(* Logix 5000 AddOnInstructionDefinition export SIKO_AP10T; software revision 19.01 *)

ADD_ON_INSTRUCTION SIKO_AP10T   (* revision 5.0 1, vendor SIKO GmbH *)
// SIKO PositionLine AP10T AOI
// Revision note:
// Usable with AP10T Firmware Vers. >= 1.06
VAR_IN_OUT
   DC_OutputBuffer : SINT[10]; {required}
   DC_AbcOutputRegister : AB:ETHERNET_MODULE_SINT_314Bytes:O:0; {required}
END_VAR
VAR_INPUT
   DC_AbcStartByteOut : INT; {required}
END_VAR
VAR_IN_OUT
   DC_InputBuffer : SINT[10]; {required}
   DC_AbcInputRegister : AB:ETHERNET_MODULE_SINT_314Bytes:I:0; {required}
END_VAR
VAR_INPUT
   DC_AbcStartByteIn : INT; {required}
   nNodeId : SINT; {visible}   // Temporaray Node_address
   nSetValue1 : DINT; {visible}
   nSetValue2 : DINT; {visible}
   nParameterAdrRead1 : SINT; {visible}
   nParameterAdrRead2 : SINT; {visible}
   nParameterAdrRead3 : SINT; {visible}
   bcStartRead : BOOL; {visible}
   bcStartWrite : BOOL; {visible}
   bcStartCopy : BOOL; {visible}
   bcResetCounterActivity : BOOL; {visible}
END_VAR
VAR_OUTPUT
   nCounterRead : INT; {access Read Only, visible}
   nCounterWrite : INT; {access Read Only, visible}
   nCounterCopy : INT; {access Read Only, visible}
   nErrorCode1 : SINT; {access Read Only, visible}
   nErrorCode2 : SINT; {access Read Only, visible}
   p00_NodeAddress_r : SINT; {access Read Only, visible}   // Parmeter: 0x00
END_VAR
VAR_INPUT
   p00_NodeAddress_w : SINT; {visible}   // Parmeter: 0x00
END_VAR
VAR_OUTPUT
   p01_Baudrate_r : SINT; {access Read Only}   // Parmeter: 0x01
END_VAR
VAR_INPUT
   p01_Baudrate_w : SINT;   // Parmeter: 0x01
END_VAR
VAR_OUTPUT
   p02_BusTimeout_r : SINT; {access Read Only}   // Parmeter: 0x02
END_VAR
VAR_INPUT
   p02_BusTimeout_w : SINT;   // Parmeter: 0x02
END_VAR
VAR_OUTPUT
   p03_ReplyWriteSetPoint_r : SINT;   // Parmeter: 0x03
END_VAR
VAR_INPUT
   p03_ReplyWriteSetPoint_w : SINT; {access Read Only}   // Parmeter: 0x03
END_VAR
VAR_OUTPUT
   p04_EnableKeysTime_r : SINT; {access Read Only}   // Parmeter: 0x04
END_VAR
VAR_INPUT
   p04_EnableKeysTime_w : SINT;   // Parmeter: 0x04
END_VAR
VAR_OUTPUT
   p05_KeyFunctionEnable1Calibrate_r : SINT; {access Read Only}   // Parmeter: 0x05
END_VAR
VAR_INPUT
   p05_KeyFunctionEnable1Calibrate_w : SINT;   // Parmeter: 0x05
   p06_LedFlashing_w : SINT;   // Parmeter: 0x06
END_VAR
VAR_OUTPUT
   p06_LedFlashing_r : SINT; {access Read Only}   // Parmeter: 0x06
   p08_Led2Red_r : SINT; {access Read Only}   // Parmeter: 0x08
END_VAR
VAR_INPUT
   p08_Led2Red_w : SINT;   // Parmeter: 0x08
END_VAR
VAR_OUTPUT
   p07_Led3Green_r : SINT; {access Read Only}   // Parmeter: 0x07
END_VAR
VAR_INPUT
   p07_Led3Green_w : SINT;   // Parmeter: 0x07
END_VAR
VAR_OUTPUT
   p09_Led1Green_r : SINT; {access Read Only}   // Parmeter: 0x09
END_VAR
VAR_INPUT
   p09_Led1Green_w : SINT;   // Parmeter: 0x09
END_VAR
VAR_OUTPUT
   p0A_DecimalPlaces_r : SINT; {access Read Only}   // Parmeter: 0x0A
END_VAR
VAR_INPUT
   p0A_DecimalPlaces_w : SINT;   // Parmeter: 0x0A
END_VAR
VAR_OUTPUT
   p0D_DisplayOrientation_r : SINT; {access Read Only}   // Parmeter: 0x0D
END_VAR
VAR_INPUT
   p0D_DisplayOrientation_w : SINT;   // Parmeter: 0x0D
END_VAR
VAR_OUTPUT
   p0E_ProgrammingMode_r : SINT; {access Read Only}   // Parmeter: 0x0E
END_VAR
VAR_INPUT
   p0E_ProgrammingMode_w : SINT; {access Read Only}   // Parmeter: 0x0E
END_VAR
VAR_OUTPUT
   p39_Led4Red_r : SINT; {access Read Only}   // Parmeter: 0x39
END_VAR
VAR_INPUT
   p39_Led4Red_w : SINT;   // Parmeter: 0x39
END_VAR
VAR_OUTPUT
   p3A_LcdBacklightFlashing_r : SINT; {access Read Only}   // Parmeter: 0x3A
END_VAR
VAR_INPUT
   p3A_LcdBacklightFlashing_w : SINT;   // Parmeter: 0x3A
END_VAR
VAR_OUTPUT
   p3B_LcdBacklightWhite_r : SINT; {access Read Only}   // Parmeter: 0x3B
END_VAR
VAR_INPUT
   p3B_LcdBacklightWhite_w : SINT;   // Parmeter: 0x3B
END_VAR
VAR_OUTPUT
   p3C_LcdBacklightRed_r : SINT; {access Read Only}   // Parmeter: 0x3C
END_VAR
VAR_INPUT
   p3C_LcdBacklightRed_w : SINT;   // Parmeter: 0x3C
END_VAR
VAR_OUTPUT
   p3D_KeyFunctionEnable3Config_r : SINT; {access Read Only}   // Parmeter: 0x3D
END_VAR
VAR_INPUT
   p3D_KeyFunctionEnable3Config_w : SINT;   // Parmeter: 0x3D
END_VAR
VAR_OUTPUT
   p3E_AcknowledgementSettings_r : SINT; {access Read Only}   // Parmeter: 0x3E
END_VAR
VAR_INPUT
   p3E_AcknowledgementSettings_w : SINT;   // Parmeter: 0x3E
END_VAR
VAR_OUTPUT
   p65_DeviceCode_r : INT; {access Read Only}   // Parmeter: 0x65
   p67_SoftwareVersion_r : INT; {access Read Only}   // Parmeter: 0x67
   p80_NumberOfErrorsRecorded_r : SINT; {access Read Only}   // Parmeter: 0x80
   p81_Error01_r : SINT; {access Read Only}   // Parmeter: 0x81
   p82_Error02_r : SINT; {access Read Only}   // Parmeter: 0x82
   p83_Error03_r : SINT; {access Read Only}   // Parmeter: 0x83
   p84_Error04_r : SINT; {access Read Only}   // Parmeter: 0x84
   p85_Error05_r : SINT; {access Read Only}   // Parmeter: 0x85
   p86_Error06_r : SINT; {access Read Only}   // Parmeter: 0x86
   p87_Error07_r : SINT; {access Read Only}   // Parmeter: 0x87
   p88_Error08_r : SINT; {access Read Only}   // Parmeter: 0x88
   p89_Error09_r : SINT; {access Read Only}   // Parmeter: 0x89
   p8A_Error10_r : SINT; {access Read Only}   // Parmeter: 0x8A
   p96_InputErrors_00_r : INT; {access Read Only}   // Parmeter: 0x96
   p96_InputErrors_01_r : INT; {access Read Only}   // Parmeter: 0x96_Sub1
   p96_InputErrors_02_r : INT; {access Read Only}   // Parmeter: 0x96_Sub2
   p96_InputErrors_03_r : INT; {access Read Only}   // Parmeter: 0x96_Sub3
   p96_InputErrors_04_r : INT; {access Read Only}   // Parmeter: 0x96_Sub4
   p96_InputErrors_05_r : INT; {access Read Only}   // Parmeter: 0x96_Sub5
   p96_InputErrors_06_r : INT; {access Read Only}   // Parmeter: 0x96_Sub6
   p96_InputErrors_07_r : INT; {access Read Only}   // Parmeter: 0x96_Sub7
   p96_InputErrors_08_r : INT; {access Read Only}   // Parmeter: 0x96_Sub8
   p96_InputErrors_09_r : INT; {access Read Only}   // Parmeter: 0x96_Sub9
   p96_InputErrors_10_r : INT; {access Read Only}   // Parmeter: 0x96_Sub10
END_VAR
VAR_INPUT
   pA0_SystemCommand_w : SINT;   // Parmeter: 0xA0
   pA8_ProgrammingModeOnOff_w : SINT;   // Parmeter: 0xA8
END_VAR
VAR_OUTPUT
   pD0_ResponseDelay_r : SINT; {access Read Only}   // Parmeter: 0xD0
END_VAR
VAR_INPUT
   pD0_ResponseDelay_w : SINT;   // Parmeter: 0xD0
   pD2_AutoIdAssignment_w : SINT;   // Parmeter: 0xD2
END_VAR
VAR_OUTPUT
   pFA_SystemStatusword_r : INT; {access Read Only}   // Parmeter: 0xFA
   pFB_SetPoint1_r : DINT; {access Read Only}   // Parmeter: 0xFB
   pFF_SetPoint2_r : DINT; {access Read Only}   // Parmeter: 0xFF
END_VAR
VAR_INPUT
   bc02_ValidityOfSetpoint1 : BOOL;
   bc03_DisplayRange : BOOL;
   bc05_ErrorAcknowledgment : BOOL;
   bc06_AcknowledgementOfSetpoint2 : BOOL;
   bc07_DataIdentifier : BOOL;
   bc09_ValidityOfSetpoint2 : BOOL;
   bc10_AcknowledgementOfSetpoint1 : BOOL;
   bc11_Led1GreenLeft : BOOL;
   bc12_Led3GreenRight : BOOL;
   bc13_Led4RedRight : BOOL;
   bc14_Led2RedLeft : BOOL;
   bc15_LedBlinking : BOOL;
END_VAR
VAR_OUTPUT
   bs02_ValiditySetpoint1 : BOOL; {access Read Only}
   bs03_AcknowledgementOfSetpoint2 : BOOL; {access Read Only}
   bs05_AcknowledgementOfSetpoint1 : BOOL; {access Read Only}
   bs06_Deviation : BOOL; {access Read Only}
   bs07_DeviceError : BOOL; {access Read Only}
   bs08_ButtonFront : BOOL; {access Read Only}
   bs09_DataIdentifier : BOOL; {access Read Only}
   bs10_ValiditySetpoint2 : BOOL;
   bs13_ButtonLeft : BOOL; {access Read Only}
   bs14_ButtonStar : BOOL; {access Read Only}
   bs15_ButtonUp : BOOL; {access Read Only}
   bsDone : BOOL; {access Read Only, visible}
   bsBusy : BOOL; {access Read Only, visible}
   bsFaultDataReceive : BOOL; {access Read Only, visible}
   bsComTimeout : BOOL; {access Read Only, visible}
   bsGeneralError : BOOL; {access Read Only, visible}
END_VAR
VAR
   vnTriggerTx : SINT; {access None}
   vnCounterToggle : SINT; {access None}
   vnTriggerRx : SINT; {access None}
   vnParameterAdrReceive : INT; {access None}
   vnParameterAdrSend : INT; {access None}
   vnParameterDataReceive : DINT; {access None}
   vnParameterDataSend : DINT; {access None}
   vbRefresh : BOOL; {access None}
   vbOsrWrite : BOOL; {access None}
   vbOsrRead : BOOL; {access None}
   vnOutputDataOffset : DINT; {access None}
   vnDcOutputBufferTemp : DINT; {access None}
   vnDcInputBufferTemp : DINT; {access None}
   vbOsrCopy : BOOL; {access None}
   SN5_ABC : FBD_TIMER; {access None}
END_VAR

ROUTINE Logic   (* structured text *)
   ///////////////////////////////////////////////////////////////////////////////////////////////
   // Name:	SIKO_AP10T
   ///////////////////////////////////////////////////////////////////////////////////////////////
   // Version history
   ///////////////////////////////////////////////////////////////////////////////////////////////
   // Date        | Version  | created under          	| Author    		| Remark
   // dd.mm.yyyy  | 		  |							|					|
   // -----------------------------------------------------------------------------------
   // 07.09.2015  | 5.0.1    | V19.01.00 (CPR 9 SR 3)  | SIKO GmbH / SC 	| basic version
   ///////////////////////////////////////////////////////////////////////////////////////////////
   
   ///////////////////////////////////////////////////////////////////////////////////////////////
   // Init at first scan
   //
   IF s:fs THEN
   	bcStartRead :=0;
   	bcStartWrite :=0;
   	bcStartCopy :=0;
   	nCounterCopy := 0;
   	nCounterWrite := 0;
   	nCounterRead := 0;
   	vnCounterToggle := 0;
   	bcResetCounterActivity := 0;
   END_IF;
   
   ///////////////////////////////////////////////////////////////////////////////////////////////
   // read inputs synchonous
   //
   CPS(DC_AbcInputRegister.data[DC_AbcStartByteIn] , DC_InputBuffer[0],10); // read from ABC
   
   ///////////////////////////////////////////////////////////////////////////////////////////////
   // input byte swop to parameter data and format transfer vnParameterAdrReceive
   //
   cop (DC_InputBuffer[5], vnDcInputBufferTemp, 1);					//Data Type Conversion
   swpb (vnDcInputBufferTemp, Reverse, vnParameterDataReceive);
   
   vnParameterAdrReceive := 16#00ff and DC_InputBuffer[2];
   
   ///////////////////////////////////////////////////////////////////////////////////////////////
   // New telegram arrived in time
   //
   SN5_ABC.Pre := (p02_BusTimeout_r * 100) + 500;							// 2000 milliseconds
   SN5_ABC.Reset := vnTriggerRx <> DC_InputBuffer[9];
   SN5_ABC.TimerEnable := vnTriggerRx = DC_InputBuffer[9];
   RTOR(SN5_ABC);
   bsComTimeout := SN5_ABC.DN;
   
   vnTriggerRx:= DC_InputBuffer[9]; // Trigger received
   
   ///////////////////////////////////////////////////////////////////////////////////////////////
   // Telegram acknowledge checked for bad reply
   //
   if vnParameterAdrReceive = 253
   then
   	bsFaultDataReceive := 1;
   	nErrorCode1 := DC_InputBuffer[8];
   	nErrorCode2 := DC_InputBuffer[7];
   
   else
   	bsFaultDataReceive := 0;
   	nErrorCode1 := 0;
   	nErrorCode2 := 0;
   end_if;
   
   
   ///////////////////////////////////////////////////////////////////////////////////////////////
   // Request (Read/Write) successful
   //
   if DC_OutputBuffer[2] = DC_InputBuffer[2] and not bsFaultDataReceive
   then
   	if nCounterRead <> 0
   	then
   		if vnParameterAdrReceive = 150							// check for parameter 0x96 Input Errors and Indexrutine
   		then
   			if DC_OutputBuffer[5] = DC_InputBuffer[5]			// check for Index: DataSend = DataReceive
   			then
   				nCounterRead := nCounterRead + 1;
   			end_if;
   		else
   			nCounterRead := nCounterRead + 1;
   		end_if;
   	end_if;
   	if nCounterWrite <> 0
   	then
   		nCounterWrite := nCounterWrite + 1;
   	end_if;
   end_if;
   
   ///////////////////////////////////////////////////////////////////////////////////////////////
   // Control word
   //
   DC_OutputBuffer[4].0 := 0;
   DC_OutputBuffer[4].1 := 0;
   DC_OutputBuffer[4].2 := bc02_ValidityOfSetpoint1;                // Validity of setpoint1; 0=invalid; 1=valid
   DC_OutputBuffer[4].3 := bc03_DisplayRange;                       // Display range full
   DC_OutputBuffer[4].4 := 0;
   DC_OutputBuffer[4].5 := bc05_ErrorAcknowledgment;                // Acknowledged
   DC_OutputBuffer[4].6 := bc06_AcknowledgementOfSetpoint2;         // Acknowledgment Set Value2
   DC_OutputBuffer[4].7 := bc07_DataIdentifier;                     // Data format, Number / ASCII-String
   DC_OutputBuffer[3].0 := 0;
   DC_OutputBuffer[3].1 := bc09_ValidityOfSetpoint2;                // Validity of setpoint2
   DC_OutputBuffer[3].2 := bc10_AcknowledgementOfSetpoint1;         // Acknowledgment Set Value2
   DC_OutputBuffer[3].3 := bc11_Led1GreenLeft;                      // LED1 green left
   DC_OutputBuffer[3].4 := bc12_Led3GreenRight;                     // LED3 green right
   DC_OutputBuffer[3].5 := bc13_Led4RedRight;                       // LED4 red right
   DC_OutputBuffer[3].6 := bc14_Led2RedLeft;                        // LED2 red left
   DC_OutputBuffer[3].7 := bc15_LedBlinking;                        // LED blinking
   
   ///////////////////////////////////////////////////////////////////////////////////////////////
   // Start Read
   //
   IF (bcStartRead or vbRefresh) AND (nCounterRead = 0) AND (nCounterWrite = 0) AND (nCounterCopy = 0)  AND NOT vbOsrRead
   THEN
   	nCounterRead := 1;
   	nCounterWrite := 0;
   	nCounterCopy := 0;
   	vbRefresh := 0;
   	vbOsrRead := 1;
   END_IF;
   IF NOT bcStartRead and vbOsrRead
   THEN
   	vbOsrRead := 0;
   END_IF;
   
   ///////////////////////////////////////////////////////////////////////////////////////////////
   // Start Write
   //
   IF bcStartWrite AND (nCounterRead = 0) AND (nCounterWrite = 0) AND (nCounterCopy = 0) AND NOT vbOsrWrite
   THEN
   	nCounterWrite := 1;
   	nCounterRead := 0;
   	nCounterCopy := 0;
   	vbOsrWrite := 1;
   END_IF;
   IF NOT bcStartWrite and vbOsrWrite
   THEN
   	vbOsrWrite := 0;
   END_IF;
   
   ///////////////////////////////////////////////////////////////////////////////////////////////
   // copy read to write parameters
   //
   IF bcStartCopy AND (nCounterRead = 0) AND (nCounterWrite = 0) AND (nCounterCopy = 0) AND NOT vbOsrCopy
   THEN
   	nCounterCopy := 1;
   	nCounterWrite := 0;
   	nCounterRead := 0;
   	vbOsrCopy := 1;
   END_IF;
   IF NOT bcStartCopy and vbOsrCopy
   THEN
   	vbOsrCopy := 0;
   END_IF;
   
   ///////////////////////////////////////////////////////////////////////////////////////////////
   // reset counter (nCounter...) and activity (bcStart...)
   //
   IF bcResetCounterActivity
   THEN
   	bcStartRead :=0;
   	bcStartWrite :=0;
   	bcStartCopy :=0;
   	nCounterCopy := 0;
   	nCounterWrite := 0;
   	nCounterRead := 0;
   	vnCounterToggle := 0;
   	bcResetCounterActivity := 0;
   END_IF;
   
   ///////////////////////////////////////////////////////////////////////////////////////////////
   // Parameter request
   //
   if nCounterRead > 0
   	then
   	DC_OutputBuffer[0] := 0;
   	vnParameterDataSend := 0;
   	CASE nCounterRead OF
   	1: //0x00 Note address
   	    vnParameterAdrSend := 0;
   	2: //0x01 Baud rate
   		vnParameterAdrSend := 1;
   	3: //0x02 Bus Timeout
         	vnParameterAdrSend := 2;
   	4: //0x03 Response parameter to a setpoint write access
         	vnParameterAdrSend := 3;
   	5: //0x04 Keys enable time: Configuration start delay
         	vnParameterAdrSend := 4;
   	6: //0x05 Key function enable1: Calibration enable
         	vnParameterAdrSend := 5;
   	7: //0x06 LED flashing
         	vnParameterAdrSend := 6;
   	8: //0x07 LED3 (green right)
         	vnParameterAdrSend := 7;
   	9: //0x08 LED2 (red left)
         	vnParameterAdrSend := 8;
   	10: //0x09 LED1 (green left)
         	vnParameterAdrSend := 9;
   	11: //0x0A Decimal places
         	vnParameterAdrSend := 10;
   	12: //0x0D Display orientation
         	vnParameterAdrSend := 13;
   	13: //0x0E Configuration programming mode
         	vnParameterAdrSend := 14;
   	14: //0x39 LED4 (red right)
         	vnParameterAdrSend := 57;
   	15: //0x3A LCD backlight flashing
         	vnParameterAdrSend := 58;
   	16: //0x3B LCD backlight white
         	vnParameterAdrSend := 59;
   	17: //0x3C LCD backlight red
         	vnParameterAdrSend := 60;
   	18: //0x3D Key function enable3: Configuration enable via keyboard
         	vnParameterAdrSend := 61;
   	19: //0x3E Acknowledgement settings
         	vnParameterAdrSend := 62;
   	20: //0x65 Device identification
         	vnParameterAdrSend := 101;
   	21: //0x67 Software version
         	vnParameterAdrSend := 103;
   	22: //0x80 Number of errors
         	vnParameterAdrSend := 128;
   	23: //0x81 Error 01
         	vnParameterAdrSend := 129;
   	24: //0x82 Error 02
         	vnParameterAdrSend := 130;
   	25: //0x83 Error 03
         	vnParameterAdrSend := 131;
   	26: //0x84 Error 04
         	vnParameterAdrSend := 132;
   	27: //0x85 Error 05
         	vnParameterAdrSend := 133;
   	28: //0x86 Error 06
         	vnParameterAdrSend := 134;
   	29: //0x87 Error 07
         	vnParameterAdrSend := 135;
   	30: //0x88 Error 08
         	vnParameterAdrSend := 136;
   	31: //0x89 Error 09
         	vnParameterAdrSend := 137;
   	32: //0x8A Error 10
         	vnParameterAdrSend := 138;
   	33: //0x96 Input Errors
   		vnParameterAdrSend := 150;
   	34: //0x96_1 Input Errors Index 1
   		vnParameterAdrSend := 150;
   		vnParameterDataSend := 16#01000000;
   	35: //0x96_2 Input Errors Index 2
   		vnParameterAdrSend := 150;
   		vnParameterDataSend := 16#02000000;
   	36: //0x96_3 Input Errors Index 3
   		vnParameterAdrSend := 150;
   		vnParameterDataSend := 16#03000000;
   	37: //0x96_4 Input Errors Index 4
   		vnParameterAdrSend := 150;
   		vnParameterDataSend := 16#04000000;
   	38: //0x96_5 Input Errors Index 5
   		vnParameterAdrSend := 150;
   		vnParameterDataSend := 16#05000000;
   	39: //0x96_6 Input Errors Index 6
   		vnParameterAdrSend := 150;
   		vnParameterDataSend := 16#06000000;
   	40: //0x96_7 Input Errors Index 7
   		vnParameterAdrSend := 150;
   		vnParameterDataSend := 16#07000000;
   	41: //0x96_8 Input Errors Index 8
   		vnParameterAdrSend := 150;
   		vnParameterDataSend := 16#08000000;
   	42: //0x96_9 Input Errors Index 9
   		vnParameterAdrSend := 150;
   		vnParameterDataSend := 16#09000000;
   	43: //0x96_10 Input Errors Index 10
   		vnParameterAdrSend := 150;
   		vnParameterDataSend := 16#0A000000;
   	44: //0xD0 Response delay
         	vnParameterAdrSend := 208;
   	45: //0xFA System Status word
         	vnParameterAdrSend := 250;
   	46: //0xFB Setpoint1
         	vnParameterAdrSend := 251;
   	47: //0xFF Setpoint2
         	vnParameterAdrSend := 255;
   	48: // Parameter read completed
   		nCounterRead := 0;
     	END_CASE;
   end_if;
   
   ///////////////////////////////////////////////////////////////////////////////////////////////
   // Parameter Settings
   //
   if nCounterWrite > 0
   	then
   	DC_OutputBuffer[0] := 1;
   	CASE nCounterWrite OF
   	1: //Programming mode
   		IF pA8_ProgrammingModeOnOff_w >= 0 and pA8_ProgrammingModeOnOff_w <= 1
   		THEN
   	      	vnParameterAdrSend := 168;
   			vnParameterDataSend:= pA8_ProgrammingModeOnOff_w;
   		END_IF;
   	2: //Note address
   		IF p00_NodeAddress_w <> p00_NodeAddress_r or bsFaultDataReceive
   		THEN
   	      	vnParameterAdrSend := 0;
   			vnParameterDataSend:= p00_NodeAddress_w;
   		END_IF;
   	3: //Baudrate
   		IF p01_Baudrate_w <> p01_Baudrate_r or bsFaultDataReceive
   		THEN
   	      	vnParameterAdrSend := 1;
   			vnParameterDataSend:= p01_Baudrate_w;
   		END_IF;
   	4: //Bus Timeout
   		IF p02_BusTimeout_w <> p02_BusTimeout_r or bsFaultDataReceive
   		THEN
   	      	vnParameterAdrSend := 2;
   			vnParameterDataSend:= p02_BusTimeout_w;
   		END_IF;
   	5: //Response parameter to a setpoint write access
   		IF p03_ReplyWriteSetPoint_w <> p03_ReplyWriteSetPoint_r or bsFaultDataReceive
   		THEN
   	      	vnParameterAdrSend := 3;
   			vnParameterDataSend:= p03_ReplyWriteSetPoint_w;
   		END_IF;
   	6: ///Keys enable time: Configuration start delay
   		IF p04_EnableKeysTime_w <> p04_EnableKeysTime_r or bsFaultDataReceive
   		THEN
   	      	vnParameterAdrSend := 4;
   			vnParameterDataSend:= p04_EnableKeysTime_w;
   		END_IF;
   	7: //Key function enable1: Calibration enable
   		IF p05_KeyFunctionEnable1Calibrate_w <> p05_KeyFunctionEnable1Calibrate_r or bsFaultDataReceive
   		THEN
   	      	vnParameterAdrSend := 5;
   			vnParameterDataSend:= p05_KeyFunctionEnable1Calibrate_w;
   		END_IF;
   	8: //LED flashing
   		IF p06_LedFlashing_w <> p06_LedFlashing_r or bsFaultDataReceive
   		THEN
   	      	vnParameterAdrSend := 6;
   			vnParameterDataSend:= p06_LedFlashing_w;
   		END_IF;
   	9: //LED3 (green right)
   		IF p07_Led3Green_w <> p07_Led3Green_r or bsFaultDataReceive
   		THEN
   	      	vnParameterAdrSend := 7;
   			vnParameterDataSend:= p07_Led3Green_w;
   		END_IF;
   	10: //LED2 (red left)
   		IF p08_Led2Red_w <> p08_Led2Red_r or bsFaultDataReceive
   		THEN
   	      	vnParameterAdrSend := 8;
   			vnParameterDataSend:= p08_Led2Red_w;
   		END_IF;
   	11: //LED1 (green left)
   		IF p09_Led1Green_w <> p09_Led1Green_r or bsFaultDataReceive
   		THEN
   	      	vnParameterAdrSend := 9;
   			vnParameterDataSend:= p09_Led1Green_w;
   		END_IF;
   	12: //Decimal places
   		IF p0A_DecimalPlaces_w <> p0A_DecimalPlaces_r or bsFaultDataReceive
   		THEN
   	      	vnParameterAdrSend := 10;
   			vnParameterDataSend := p0A_DecimalPlaces_w;
   		END_IF;
   	13: //Display orientation
   		IF p0D_DisplayOrientation_w <> p0D_DisplayOrientation_r or bsFaultDataReceive
   		THEN
   	      	vnParameterAdrSend := 13;
   			vnParameterDataSend:= p0D_DisplayOrientation_w;
   		END_IF;
   	14: //Configuration programming mode
   		IF p0E_ProgrammingMode_w <> p0E_ProgrammingMode_r or bsFaultDataReceive
   		THEN
   	      	vnParameterAdrSend := 14;
   			vnParameterDataSend:= p0E_ProgrammingMode_w;
   		END_IF;
   	15: //LED4 (red right)
   		IF p39_Led4Red_w <> p39_Led4Red_r or bsFaultDataReceive
   		THEN
   	      	vnParameterAdrSend := 57;
   			vnParameterDataSend:= p39_Led4Red_w;
   		END_IF;
   	16: //LCD backlight flashing
   		IF p3A_LcdBacklightFlashing_w <> p3A_LcdBacklightFlashing_r or bsFaultDataReceive
   		THEN
   	      	vnParameterAdrSend := 58;
   			vnParameterDataSend:= p3A_LcdBacklightFlashing_w;
   		END_IF;
   	17: //LCD backlight white
   		IF p3B_LcdBacklightWhite_w <> p3B_LcdBacklightWhite_r or bsFaultDataReceive
   		THEN
   	      	vnParameterAdrSend := 59;
   			vnParameterDataSend:= p3B_LcdBacklightWhite_w;
   		END_IF;
   	18: //LCD backlight red
   		IF p3C_LcdBacklightRed_w <> p3C_LcdBacklightRed_r or bsFaultDataReceive
   		THEN
   	      	vnParameterAdrSend := 60;
   			vnParameterDataSend:= p3C_LcdBacklightRed_w;
   		END_IF;
   	19: //Key function enable3: Configuration enable via keyboard
   		IF p3D_KeyFunctionEnable3Config_w <> p3D_KeyFunctionEnable3Config_r or bsFaultDataReceive
   		THEN
   	      	vnParameterAdrSend := 61;
   			vnParameterDataSend:= p3D_KeyFunctionEnable3Config_w;
   		END_IF;
   	20: //Acknowledgement settings
   		IF p3E_AcknowledgementSettings_w <> p3E_AcknowledgementSettings_r or bsFaultDataReceive
   		THEN
   	      	vnParameterAdrSend := 62;
   			vnParameterDataSend:= p3E_AcknowledgementSettings_w;
   		END_IF;
   	21: //Response delay
   		IF pD0_ResponseDelay_w <> pD0_ResponseDelay_r or bsFaultDataReceive
   		THEN
   	      	vnParameterAdrSend := 208;
   			vnParameterDataSend:= pD0_ResponseDelay_w;
   		END_IF;
   	22: //Auto-ID assignment
   		IF pD2_AutoIdAssignment_w >= 1 and pD2_AutoIdAssignment_w <= 31 and nNodeId = 31
   		THEN
   	      	vnParameterAdrSend := 210;
   			vnParameterDataSend:= pD2_AutoIdAssignment_w;
   		END_IF;
   	23: //S-Befehl
   		IF pA0_SystemCommand_w >= 1 and pA0_SystemCommand_w <= 9 // check, if value is between 1 and 9
   		THEN
   	      	vnParameterAdrSend := 160;
   			vnParameterDataSend:= pA0_SystemCommand_w;
   			vbRefresh := 1;
   		END_IF;
   	24:	//Write complete start refresh if S-Command
   		nCounterWrite := 0;
   
   	END_CASE;
   end_if;
   ///////////////////////////////////////////////////////////////////////////////////////////////
   // Read/Write standard values and three free parameters if parameter read/write inactive
   //
   if (nCounterRead = 0) and (nCounterWrite = 0)
   then
   	if (vnCounterToggle < 1) or (vnCounterToggle > 5)
   	then
   		vnCounterToggle := 1;
   	end_if;
   
   	CASE vnCounterToggle OF
   	1:	//check SetValue and transmit
   		DC_OutputBuffer[0] := 1;
      		vnParameterAdrSend := 251;
   		vnParameterDataSend := nSetValue1;
   
   		if (vnParameterAdrReceive = 251) and DC_InputBuffer[0] = 1
   		then
   			vnCounterToggle := vnCounterToggle + 1;
   		end_if;
   
   	2:	//check SetValue and transmit
   		DC_OutputBuffer[0] := 1;
      		vnParameterAdrSend := 255;
   		vnParameterDataSend := nSetValue2;
   
   		if (vnParameterAdrReceive = 255) and DC_InputBuffer[0] = 1
   		then
   			vnCounterToggle := vnCounterToggle + 1;
   		end_if;
   
   	3:	//vnParameterAdrRead1
   		if ((16#00ff and nParameterAdrRead1) <= 250)
   		then
   			DC_OutputBuffer[0] := 0;
   			vnParameterAdrSend := nParameterAdrRead1;
   			vnParameterDataSend := 0;
   		else
   			vnCounterToggle := vnCounterToggle + 1;
   		end_if;
   
   		if vnParameterAdrReceive = (16#00ff and nParameterAdrRead1) and DC_InputBuffer[0] = 0
   		then
   			vnCounterToggle := vnCounterToggle + 1;
   		end_if;
   
   	4:	//vnParameterAdrRead2
   		if ((16#00ff and nParameterAdrRead2) <= 250)
   		then
   			DC_OutputBuffer[0] := 0;
   			vnParameterAdrSend := nParameterAdrRead2;
   			vnParameterDataSend := 0;
   		else
   			vnCounterToggle := vnCounterToggle + 1;
   		end_if;
   
   		if vnParameterAdrReceive = (16#00ff and nParameterAdrRead2) and DC_InputBuffer[0] = 0
   		then
   			vnCounterToggle := vnCounterToggle + 1;
   		end_if;
   
   	5:	//vnParameterAdrRead3
   		if ((16#00ff and nParameterAdrRead3) <= 250)
   		then
   			DC_OutputBuffer[0] := 0;
   			vnParameterAdrSend := nParameterAdrRead3;
   			vnParameterDataSend := 0;
   		else
   			vnCounterToggle := vnCounterToggle + 1;
   		end_if;
   
   		if vnParameterAdrReceive = (16#00ff and nParameterAdrRead3) and DC_InputBuffer[0] = 0
   		then
   			vnCounterToggle := vnCounterToggle + 1;
   		end_if;
   
   	END_CASE;
   else
   	vnCounterToggle := 0;
   end_if;
   
   ///////////////////////////////////////////////////////////////////////////////////////////////
   // Because of Arthmetic overflow
   //
   if vnTriggerTx >= 127
   then
    vnTriggerTx := -128;
   end_if;
   vnTriggerTx := vnTriggerTx + 1; // ABC Update mode: Change of state on trigger
   
   ///////////////////////////////////////////////////////////////////////////////////////////////
   // Telegram will be completed
   //
   DC_OutputBuffer[1] := nNodeId;
   DC_OutputBuffer[2] := 16#00ff and vnParameterAdrSend;
   DC_OutputBuffer[9] := vnTriggerTx; // Trigger transmit
   
   ///////////////////////////////////////////////////////////////////////////////////////////////
   ///////////////////////////////////////////////////////////////////////////////////////////////
   
   ///////////////////////////////////////////////////////////////////////////////////////////////
   // Confirmation of Parameter request / Parameter Settings
   //
   IF DC_InputBuffer[1] = nNodeId //Check node address
   THEN
   //	vnParameterAdrReceive := 16#00ff and DC_InputBuffer[2]; //Check command acknowledgment
   	CASE vnParameterAdrReceive OF
   		251: //Setpoint1
   			COP (vnParameterDataReceive,pFB_SetPoint1_r,1);
   		255: //Setpoint2
   			COP (vnParameterDataReceive,pFF_SetPoint2_r,1);
   		0: //Note address
   			COP (vnParameterDataReceive,p00_NodeAddress_r,1);
   		1: //Baudrate
   			COP (vnParameterDataReceive,p01_Baudrate_r,1);
   		2: //Bus Timeout
   			COP (vnParameterDataReceive,p02_BusTimeout_r,1);
   		3: //Response parameter to a setpoint write access
   			COP (vnParameterDataReceive,p03_ReplyWriteSetPoint_r,1);
   		4: //Keys enable time: Configuration start delay
   			COP (vnParameterDataReceive,p04_EnableKeysTime_r,1);
   		5: //Key function enable1: Calibration enable
   			COP (vnParameterDataReceive,p05_KeyFunctionEnable1Calibrate_r,1);
   		6: //LED flashing
   			COP (vnParameterDataReceive,p06_LedFlashing_r,1);
   		7: //LED3 (green right)
   			COP (vnParameterDataReceive,p07_Led3Green_r,1);
   		8: //LED2 (red left)
   			COP (vnParameterDataReceive,p08_Led2Red_r,1);
   		9: //LED1 (green left)
   			COP (vnParameterDataReceive,p09_Led1Green_r,1);
   		10: //Decimal places
   			COP (vnParameterDataReceive,p0A_DecimalPlaces_r,1);
   		13: //Display orientation
   			COP (vnParameterDataReceive,p0D_DisplayOrientation_r,1);
   		14: //Configuration programming mode
   			COP (vnParameterDataReceive,p0E_ProgrammingMode_r,1);
   		57:	//LED4 (red right)
   			COP (vnParameterDataReceive,p39_Led4Red_r,1);
   		58:	//LCD backlight flashing
   			COP (vnParameterDataReceive,p3A_LcdBacklightFlashing_r,1);
   		59:	//LCD backlight white
   			COP (vnParameterDataReceive,p3B_LcdBacklightWhite_r,1);
   		60:	//LCD backlight red
   			COP (vnParameterDataReceive,p3C_LcdBacklightRed_r,1);
   		61: //Key function enable3: Configuration enable via keyboard
   			COP (vnParameterDataReceive,p3D_KeyFunctionEnable3Config_r,1);
   		62:	//Acknowledgement settings
   			COP (vnParameterDataReceive,p3E_AcknowledgementSettings_r,1);
   		101: //Device identification
   			COP (vnParameterDataReceive,p65_DeviceCode_r,1);
   		103: //Software version
   			COP (vnParameterDataReceive,p67_SoftwareVersion_r,1);
   		128: //Number of errors
   			COP (vnParameterDataReceive,p80_NumberOfErrorsRecorded_r,1);
   		129: //Error01
   			COP (vnParameterDataReceive,p81_Error01_r,1);
   		130: //Error02
   			COP (vnParameterDataReceive,p82_Error02_r,1);
   		131: //Error03
   			COP (vnParameterDataReceive,p83_Error03_r,1);
   		132: //Error04
   			COP (vnParameterDataReceive,p84_Error04_r,1);
   		133: //Error05
   			COP (vnParameterDataReceive,p85_Error05_r,1);
   		134: //Error06
   			COP (vnParameterDataReceive,p86_Error06_r,1);
   		135: //Error07
   			COP (vnParameterDataReceive,p87_Error07_r,1);
   		136: //Error08
   			COP (vnParameterDataReceive,p88_Error08_r,1);
   		137: //Error09
   			COP (vnParameterDataReceive,p89_Error09_r,1);
   		138: //Error10
   			COP (vnParameterDataReceive,p8A_Error10_r,1);
   		150: //Input errors
   			if vnParameterDataSend = 0
   				then
   					COP (vnParameterDataReceive,p96_InputErrors_00_r,1);
   				end_if;
   			if vnParameterDataSend = 16#01000000
   				then
   					COP (vnParameterDataReceive,p96_InputErrors_01_r,1);
   				end_if;
   			if vnParameterDataSend = 16#02000000
   				then
   					COP (vnParameterDataReceive,p96_InputErrors_02_r,1);
   				end_if;
   			if vnParameterDataSend = 16#03000000
   				then
   					COP (vnParameterDataReceive,p96_InputErrors_03_r,1);
   				end_if;
   			if vnParameterDataSend = 16#04000000
   				then
   					COP (vnParameterDataReceive,p96_InputErrors_04_r,1);
   				end_if;
   			if vnParameterDataSend = 16#05000000
   				then
   					COP (vnParameterDataReceive,p96_InputErrors_05_r,1);
   				end_if;
   			if vnParameterDataSend = 16#06000000
   				then
   					COP (vnParameterDataReceive,p96_InputErrors_06_r,1);
   				end_if;
   			if vnParameterDataSend = 16#07000000
   				then
   					COP (vnParameterDataReceive,p96_InputErrors_07_r,1);
   				end_if;
   			if vnParameterDataSend = 16#08000000
   				then
   					COP (vnParameterDataReceive,p96_InputErrors_08_r,1);
   				end_if;
   			if vnParameterDataSend = 16#09000000
   				then
   					COP (vnParameterDataReceive,p96_InputErrors_09_r,1);
   				end_if;
   			if vnParameterDataSend = 16#0A000000
   				then
   					COP (vnParameterDataReceive,p96_InputErrors_10_r,1);
   				end_if;
   
   		208: //Response delay
   			COP (vnParameterDataReceive,pD0_ResponseDelay_r,1);
   		250: //System Status word
   			COP (vnParameterDataReceive,pFA_SystemStatusword_r,1);
   		END_CASE;
   END_IF;
   
   ///////////////////////////////////////////////////////////////////////////////////////////////
   // handle copy instruction
   //
   
   IF (nCounterCopy > 0)
   THEN
   	p00_NodeAddress_w := p00_NodeAddress_r;
   	p01_Baudrate_w := p01_Baudrate_r;
   	p02_BusTimeout_w := p02_BusTimeout_r;
   	p03_ReplyWriteSetPoint_w := p03_ReplyWriteSetPoint_r;
   	p04_EnableKeysTime_w := p04_EnableKeysTime_r;
   	p05_KeyFunctionEnable1Calibrate_w := p05_KeyFunctionEnable1Calibrate_r;
   	p06_LedFlashing_w := p06_LedFlashing_r;
   	p07_Led3Green_w := p07_Led3Green_r;
   	p08_Led2Red_w := p08_Led2Red_r;
   	p09_Led1Green_w := p09_Led1Green_r;
   	p0A_DecimalPlaces_w := p0A_DecimalPlaces_r;
   	p0D_DisplayOrientation_w := p0D_DisplayOrientation_r;
   	p0E_ProgrammingMode_w := p0E_ProgrammingMode_r;
   	p39_Led4Red_w := p39_Led4Red_r;
   	p3A_LcdBacklightFlashing_w := p3A_LcdBacklightFlashing_r;
   	p3B_LcdBacklightWhite_w := p3B_LcdBacklightWhite_r;
   	p3C_LcdBacklightRed_w := p3C_LcdBacklightRed_r;
   	p3D_KeyFunctionEnable3Config_w := p3D_KeyFunctionEnable3Config_r;
   	p3E_AcknowledgementSettings_w := p3E_AcknowledgementSettings_r;
   	pD0_ResponseDelay_w := pD0_ResponseDelay_r;
   
   	nCounterCopy := 0;
   END_IF;
   
   ///////////////////////////////////////////////////////////////////////////////////////////////
   // Status word
   //
   // bs00_ 				 					:= DC_InputBuffer[4].0;
   // bs01_									:= DC_InputBuffer[4].1;
   bs02_ValiditySetpoint1 						:= DC_InputBuffer[4].2; //set_value1_ack
   bs03_AcknowledgementOfSetpoint2				:= DC_InputBuffer[4].3; //AcknowledgementOfSetpoint2
   // bs04_									:= DC_InputBuffer[4].4;
   bs05_AcknowledgementOfSetpoint1				:= DC_InputBuffer[4].5; //AcknowledgementOfSetpoint1
   bs06_Deviation								:= DC_InputBuffer[4].6; //deviation
   bs07_DeviceError 							:= DC_InputBuffer[4].7; //Error
   bs08_ButtonFront		 					:= DC_InputBuffer[3].0; //AV_position
   bs09_DataIdentifier							:= DC_InputBuffer[3].1; //incremental_measure
   bs10_ValiditySetpoint2          			:= DC_InputBuffer[3].2; //set_value2_ack
   // bs11_			 						:= DC_InputBuffer[3].3;
   // bs12_			           				:= DC_InputBuffer[3].4;
   bs13_ButtonLeft 							:= DC_InputBuffer[3].5; //button_left
   bs14_ButtonStar 							:= DC_InputBuffer[3].6; //button_star
   bs15_ButtonUp 								:= DC_InputBuffer[3].7; //button_up
   
   ///////////////////////////////////////////////////////////////////////////////////////////////
   // Read and Write cycle completed or inactive
   //
   if nCounterRead = 0 and nCounterWrite = 0 and nCounterCopy = 0
   then
   	bsDone := 1;
   	bsBusy :=0;
   else
   	bsDone :=0;
   	bsBusy := 1;
   end_if;
   
   ///////////////////////////////////////////////////////////////////////////////////////////////
   // Dievice or transmit error occured
   //
   if bsFaultDataReceive or bs07_DeviceError or bsComTimeout
   then
   	bsGeneralError := 1;
   	bsDone :=0;
   else
   	bsGeneralError := 0;
   end_if;
   
   ///////////////////////////////////////////////////////////////////////////////////////////////
   // parameter data byte swop to output
   //
   swpb (vnParameterDataSend, Reverse, vnDcOutputBufferTemp);
   Cop (vnDcOutputBufferTemp, DC_OutputBuffer[5], 4);					//Data Type Conversion
   
   ///////////////////////////////////////////////////////////////////////////////////////////////
   // Write outputs synchonous
   //
   CPS(DC_OutputBuffer[0],DC_AbcOutputRegister.data[DC_AbcStartByteOut+vnOutputDataOffset],10); //transmit to ABC
   
END_ROUTINE
END_ADD_ON_INSTRUCTION
